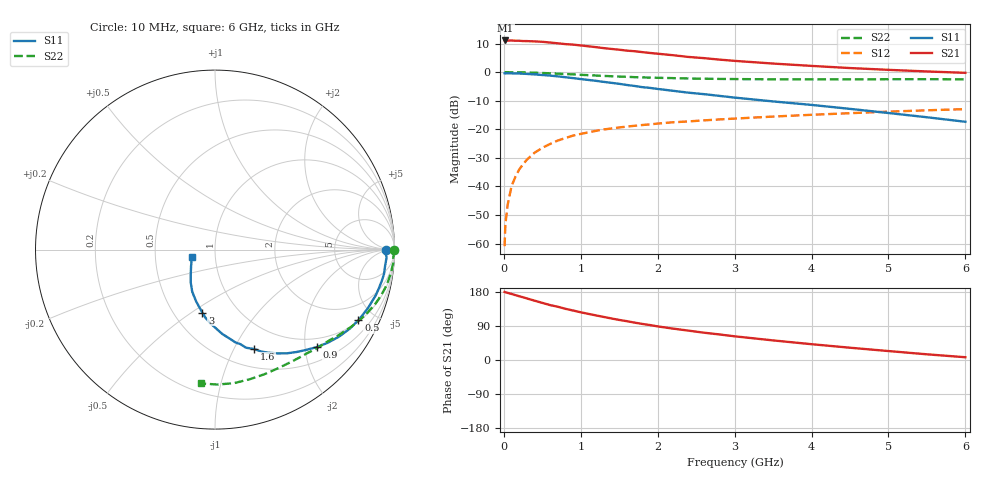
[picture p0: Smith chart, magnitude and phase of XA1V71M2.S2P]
! SIEMENS Discrete & RF Semiconductors
! BFY180
! Si NPN RF Bipolar Junction Transistor in MICRO-X
! VCE = 1.75 V  IC = 1.2 mA
! Common Emitter S-Parameters:  May  1997
# GHz  S  MA  R  50
!  f  S11  S21  S12  S22
! GHz  MAG  ANG  MAG  ANG  MAG  ANG  MAG  ANG
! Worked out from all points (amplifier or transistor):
!   36 points, 10 MHz to 6 GHz, reference 50 ohm
!   highest |S21| = 11.1 dB at 20 MHz (marker M1)
!   |S21| within 3 dB of that: start of sweep to 1.41 GHz
!   unconditionally stable (mu >= 1): 3.232 GHz to end of sweep
!   at 250 MHz: K = 0.10, MSG = 21.6 dB, |S12| = -32.3 dB
!   at 1.4 GHz: K = 0.58, MSG = 13.9 dB, |S12| = -19.7 dB
!   at 6 GHz: K = 1.08, MAG = 4.6 dB, |S12| = -12.9 dB
!   S11 on the Smith chart (normalised r, x): 10 MHz: 42, -5; 500 MHz: 1.06, -4.04; 900 MHz: 0.79, -2.26; 1.6 GHz: 0.70, -1.21; 3 GHz: 0.69, -0.55; 6 GHz: 0.77, -0.07
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0.01  0.9536 -0.3  3.562 179.6  0.0009 94.3  0.9977 -0.2
0.02  0.9478 -1.0  3.585 178.8  0.0022 88.2  0.9999 -0.7
0.05  0.9572 -2.5  3.562 177.2  0.0048 84.0  0.9967 -1.5
0.1  0.952 -5.5  3.575 174.3  0.0101 88.1  0.9935 -2.9
0.15  0.9513 -8.2  3.544 171.3  0.0147 85.5  0.9963 -4.3
0.2  0.9461 -10.4  3.54 168.2  0.0198 83.1  0.9917 -5.8
0.3  0.9314 -15.8  3.492 162.4  0.0294 79.4  0.9852 -8.6
0.5  0.891 -26.2  3.395 150.7  0.0473 72.5  0.9661 -14.0
0.6  0.8701 -30.5  3.296 145.0  0.0552 69.3  0.9536 -16.6
0.9  0.7858 -43.7  3.032 130.6  0.0775 60.7  0.9134 -23.6
1.1  0.7299 -51.4  2.832 121.7  0.0884 56.0  0.8851 -27.6
1.4  0.65 -62.2  2.546 109.6  0.1032 50.2  0.8478 -33.1
1.6  0.5955 -68.5  2.378 102.4  0.1115 47.4  0.8283 -36.3
1.8  0.5459 -74.9  2.239 95.2  0.1187 44.6  0.809 -39.4
2  0.5077 -80.0  2.101 88.7  0.1259 42.1  0.7962 -42.3
2.2  0.4717 -85.1  1.977 82.8  0.1326 39.6  0.7858 -45.2
2.6  0.4122 -93.6  1.759 72.1  0.1431 35.9  0.7671 -50.5
3  0.3585 -101.3  1.575 62.5  0.1538 32.5  0.7563 -55.6
3.5  0.3072 -110.0  1.413 51.7  0.1669 28.9  0.7489 -61.9
4.5  0.2276 -126.4  1.179 32.4  0.1913 21.6  0.7478 -75.0
5.5  0.1623 -145.3  1.028 15.0  0.2148 13.7  0.752 -89.0
6  0.1353 -162.0  0.972 7.3  0.2254 9.7  0.7498 -96.1
